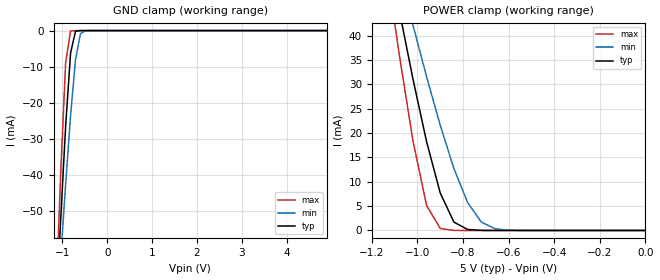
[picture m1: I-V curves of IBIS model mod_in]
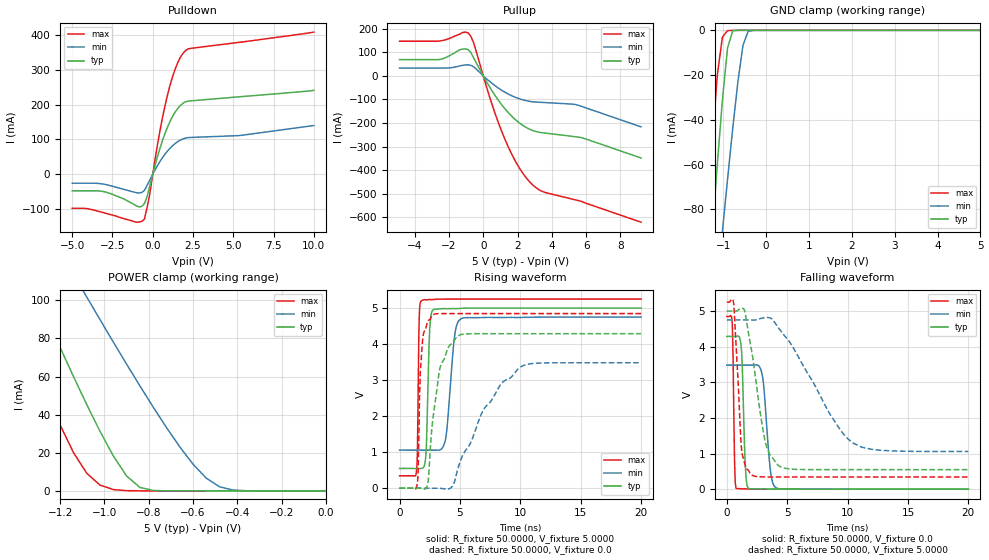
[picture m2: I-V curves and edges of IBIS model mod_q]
| IBIS (I/O, Buffer, Information, Specification) Model, officially
| electronic behavioral standard for Buffer structures of digital pins.
[IBIS ver]  4.0
[File name] 54act273_5v0_rev1.ibs
[File Rev]  1.0
[Date]   3 June 2024
[Source]   CAD & Design Services (Catania) - STMicroelectronics
[Notes]
   (Note1)  This IBIS model includes the Flat-20 package data
   (Note2)  This IBIS model has some Notes about the non-monotonicity
   of the I-V curves, but they are not indicative of problems
   inside the model;
[Disclaimer]
   Customers are solely responsible for all aspects of their
   own product designs or applications using this IBIS Model.
   STMicroelectronics assumes no liability for Custmer Designs
   and applications associated to this IBIS Model.
   In the use of this IBIS Model Customer shall not modify,
   disassemble, alter this Model in whole or in part.
   If Customers do not accept these terms, the IBIS Model
   may not be used. For any problems or modifications please
   contact STMicroelectronics (www.st.com).
[Copyright] (c) 2024 STMicroelectronics
|   Component 54ACT273
[Component] 54ACT273
[Manufacturer] STMicroelectronics
[Package]
| variable   typ   min   max
R_pkg   0.0   0.0   0.0
L_pkg   0.0H   0.0H   0.0H
C_pkg   0.0F   0.0F   0.0F
[Pin]   signal_name   model_name   R_pin   L_pin   C_pin
1   CL   mod_in   178.9m   6.2nH   1.2pF
2   Q0   mod_q   182.5m   6.3nH   1.2pF
3   D0   mod_in   114.4m   3.5nH   1.3pF
4   D1   mod_in   79.1m   2.3nH   0.9pF
5   Q1   mod_q   75.8m   2.2nH   0.8pF
6   Q2   mod_q   75.8m   2.2nH   0.8pF
7   D2   mod_in   84.5m   2.4nH   0.9pF
8   D3   mod_in   116.2m   3.6nH   1.3pF
9   Q3   mod_q   178.9m   6.2nH   1.2pF
10   GND   GND   117.4m   4.4nH   1.2pF
11   CP   mod_in   178.9m   6.2nH   1.2pF
12   Q4   mod_q   189.6m   6.6nH   1.2pF
13   D4   mod_in   125.1m   3.9nH   1.3pF
14   D5   mod_in   86.3m   2.5nH   0.9pF
15   Q5   mod_q   79.4m   2.3nH   0.8pF
16   Q6   mod_q   75.8m   2.2nH   0.8pF
17   D6   mod_in   75.6m   2.1nH   0.9pF
18   D7   mod_in   89.3m   2.7nH   1.3pF
19   Q7   mod_q   184.3m   6.4nH   1.2pF
20   VCC   POWER   118.0m   4.4nH   1.2pF
| Models and submodels in the file (2): mod_in (Input), mod_q (I/O)
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|   Model mod_in
[Model]   mod_in
Model_type Input
Vinl   =   1.500V
Vinh   =   3.500V
C_comp   0.532pF   0.404pF   0.670pF
[Temperature Range]  25.0000   0.1250k   -55.0000
[Voltage Range]   5.0000V   4.7500V   5.2500V
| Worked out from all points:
|   GND clamp passes 1 mA (typ) near -0.72 V on its own axis
|   POWER clamp passes 1 mA (typ) near -0.81 V on its own axis
[GND_clamp]
|Voltage   I(typ)   I(min)   I(max)
-5V       -1.137A    -886.9mA   -1.491A
-1.15V    -80.11mA   -84.56mA   -76mA
-1.04V    -52.42mA   -63.27mA   -39.57mA
-930mV    -26.56mA   -42.73mA   -8.977mA
-820mV    -6.248mA   -23.65mA   -92.59uA
-710mV    -202uA     -8.091mA   -269.9nA
-600mV    -2.872uA   -885uA     -788.8pA
-490mV    -39.72nA   -40.33uA   -14.69pA
4.9V      9.601pA    191.6pA    9.1pA
[POWER_clamp]
|Voltage   I(typ)   I(min)   I(max)
-4.98V    1.112A     863.1mA    1.464A
-1.14V    59.96mA    64.62mA    55.5mA
-1.08V    45.22mA    53.27mA    36.14mA
-1.02V    31.13mA    42.2mA     18.48mA
-960mV    18.22mA    31.55mA    5.125mA
-900mV    7.677mA    21.57mA    415.2uA
-840mV    1.714mA    12.69mA    18.08uA
-780mV    205.3uA    5.736mA    745.1nA
-720mV    20.39uA    1.733mA    30.64nA
-660mV    1.979uA    364.6uA    1.272nA
-600mV    191.5nA    66.12uA    64.63pA
0V        10pA       57.63pA    10.5pA
|   Model mod_q
[Model]   mod_q
Model_type I/O
Polarity   Non-Inverting
Enable   Active-High
Vinl   =   1.500V
Vinh   =   3.500V
Vmeas  =   2.500V
Rref   =   500
Cref   =   50pF
C_comp   2.925pF   2.219pF   3.850pF
[Temperature Range]  25.0000   0.1250k   -55.0000
[Voltage Range]   5.0000V   4.7500V   5.2500V
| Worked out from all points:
|   slope of the pulldown table from 0 to 0.75 V, typ, clamps not added: 6.47 ohm
|   slope of the pullup table from 0 to 0.75 V, typ, clamps not added: 8.34 ohm
|   GND clamp passes 1 mA (typ) near -0.79 V on its own axis
|   POWER clamp passes 1 mA (typ) near -0.81 V on its own axis
|   rising waveform, R_fixture 50.0000, V_fixture 5.0000: 20-80 % time 212ps typ, 522ps min, 106ps max; typ from 0.548 V to 5 V
|   rising waveform, R_fixture 50.0000, V_fixture 0.0: 20-80 % time 931ps typ, 3.22ns min, 282ps max; typ from 0 V to 4.29 V
|   falling waveform, R_fixture 50.0000, V_fixture 0.0: 20-80 % time 230ps typ, 471ps min, 123ps max; typ from 4.29 V to 0 V
|   falling waveform, R_fixture 50.0000, V_fixture 5.0000: 20-80 % time 1.18ns typ, 3.71ns min, 443ps max; typ from 5 V to 0.548 V
[Pulldown]
|Voltage   I(typ)   I(min)   I(max)
-5V       -47.76mA   -25.94mA   -98.12mA
-3.08V    -49.72mA   -28.26mA   -110.4mA
-840mV    -94.02mA   -54.15mA   -137.5mA
-520mV    -84.67mA   -46.77mA   -129.3mA
-200mV    -36.8mA    -18.22mA   -61.09mA
440mV     73.46mA    36.03mA    123.3mA
920mV     135.7mA    66.79mA    228.6mA
1.4V      179.2mA    88.62mA    303.4mA
1.72V     197.8mA    98.22mA    336.3mA
2.04V     208.1mA    103.9mA    355.6mA
5.4V      222.6mA    111.3mA    379.2mA
10V       241mA      139.8mA    408.5mA
[Pullup]
|Voltage   I(typ)   I(min)   I(max)
-4.88V    68.6mA     32.87mA    146.8mA
-2.48V    69.99mA    32.87mA    148.2mA
-1.36V    110.7mA    42mA       177.2mA
-880mV    110.9mA    46.75mA    182mA
-560mV    76.32mA    38.59mA    140.2mA
400mV     -50.52mA   -25.5mA    -96.03mA
1.2V      -133.8mA   -66.67mA   -257.5mA
2V        -193.4mA   -94.55mA   -377.6mA
2.64V     -224mA     -107.3mA   -443.9mA
3.44V     -241.1mA   -112.7mA   -489.6mA
5.36V     -257.9mA   -121.5mA   -525.3mA
9.2V      -348.1mA   -216.2mA   -620mA
[GND_clamp]
|Voltage   I(typ)   I(min)   I(max)
-5V       -1.118A    -920.1mA   -1.399A
-1.38V    -122mA     -162.2mA   -88.14mA
-1.26V    -90.61mA   -137.8mA   -51.22mA
-1.14V    -60.05mA   -113.7mA   -20.14mA
-1.02V    -31.25mA   -89.87mA   -3.05mA
-900mV    -7.839mA   -66.52mA   -145.1uA
-780mV    -258.7uA   -43.99mA   -5.698uA
-660mV    -6.646uA   -23.14mA   -226nA
-540mV    -379.1nA   -6.677mA   -9.132nA
-420mV    -27.81nA   -473.7uA   -398pA
-180mV    -283.7pA   -494.2nA   -26.46pA
5V        3.83nA     9.459nA    298.4pA
[POWER_clamp]
|Voltage   I(typ)   I(min)   I(max)
-5V       1.118A     920.1mA    1.399A
-1.44V    137.9mA    174.4mA    107.6mA
-1.38V    122mA      162.2mA    88.14mA
-1.32V    106.2mA    150mA      69.24mA
-1.2V     75.19mA    125.7mA    34.58mA
-1.08V    45.32mA    101.7mA    9.265mA
-960mV    18.36mA    78.12mA    710.8uA
-840mV    1.841mA    55.12mA    28.78uA
-660mV    6.646uA    23.14mA    226nA
-540mV    379.1nA    6.677mA    9.132nA
-420mV    27.81nA    473.7uA    398pA
0V        111.1pA    6.851nA    24.03pA
[Ramp]
| variable   typ   min   max
dV/dt_r   2.5731/0.9600n   2.0895/3.2691n   2.9081/0.3171n
dV/dt_f   2.5420/0.9550n   2.0853/3.1591n   2.8770/0.3130n
R_load = 50.0000
[Rising Waveform]
R_fixture= 50.0000
V_fixture= 5.0000
V_fixture_min= 4.7500
V_fixture_max= 5.2500
|time   V(typ)   V(min)   V(max)
0s        547.7mV    1.056V     342.4mV
1.4ns     547.7mV    1.056V     450.4mV
1.64ns    548.1mV    1.056V     4.811V
1.82ns    545.3mV    1.056V     5.205V
2.18ns    889.7mV    1.056V     5.228V
2.5ns     4.408V     1.056V     5.239V
2.8ns     4.956V     1.056V     5.239V
3.8ns     4.98V      1.343V     5.25V
5.04ns    4.992V     4.692V     5.25V
20ns      5V         4.75V      5.25V
[Rising Waveform]
R_fixture= 50.0000
V_fixture= 0.0
V_fixture_min= 0.0
V_fixture_max= 0.0
|time   V(typ)   V(min)   V(max)
0s        145.2pV    429.9pV    91.9pV
1.46ns    -21.77uV   -129.2nV   94.51mV
1.7ns     1.003mV    219.2nV    3.042V
1.88ns    -7.835mV   941.6nV    3.986V
2.38ns    206.4mV    -6.953uV   4.647V
2.78ns    1.971V     34.49uV    4.814V
3.46ns    3.457V     -7.993mV   4.847V
4.98ns    4.252V     697.2mV    4.847V
10.14ns   4.288V     3.386V     4.847V
20ns      4.288V     3.482V     4.847V
[Falling Waveform]
R_fixture= 50.0000
V_fixture= 0.0
V_fixture_min= 0.0
V_fixture_max= 0.0
|time   V(typ)   V(min)   V(max)
0s        4.288V     3.482V     4.847V
460ps     4.288V     3.482V     4.637V
640ps     4.288V     3.482V     850.4mV
760ps     4.288V     3.482V     26.67mV
1.18ns    4.053V     3.482V     9.417mV
1.54ns    628.2mV    3.482V     8.08mV
1.78ns    30.69mV    3.482V     5.73mV
2.92ns    6.482mV    3.23V      513.5uV
4.06ns    5.197mV    42.05mV    14.94uV
20ns      -24.33nV   3.42uV     180.8pV
[Falling Waveform]
R_fixture= 50.0000
V_fixture= 5.0000
V_fixture_min= 4.7500
V_fixture_max= 5.2500
|time   V(typ)   V(min)   V(max)
0s        5V         4.75V      5.25V
580ps     5V         4.75V      5.189V
1.24ns    5.084V     4.75V      1.067V
1.48ns    5.01V      4.75V      726.7mV
2.02ns    3.954V     4.75V      409.5mV
3.16ns    1.37V      4.817V     343.9mV
4.36ns    646.1mV    4.492V     342.4mV
8.56ns    547.8mV    2.096V     342.4mV
10.42ns   547.7mV    1.3V       342.4mV
20ns      547.7mV    1.056V     342.4mV
